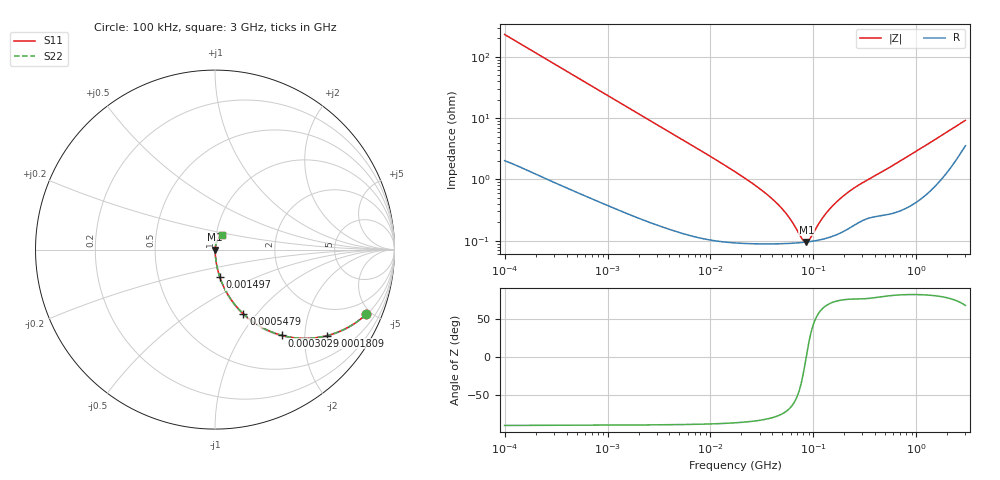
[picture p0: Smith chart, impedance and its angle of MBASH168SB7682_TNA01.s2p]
! MBASH168SB7682_TNA01  S-PARAMETER MODEL  ( Standard Model )
! Model Generated by TAIYO YUDEN Corporation (http://www.ty-top.com)
! Version 1.0
! TAIYO YUDEN Control No. 220601
! Copyright(c) 2013 TAIYO YUDEN CO.,LTD. All Rights Reserved.
! Product Description (link to TY-COMPAS)
! https://ds.yuden.co.jp/TYCOMPAS/or/detail?pn=MBASH168SB7682KTNA01&u=M
! Products Name : Multilayer Ceramic Capacitors
! Characteristics :
!  Capacitance : 6800 [pF] , Rated Voltage : 100 [V] , TCC : X7R
!  Case Size : 1.6 x 0.8 / 0.063 x 0.031 [mm/inch] , Thickness : 0.8 / 0.031 [mm/inch]
!  (Conditions: Temperature = 25 [degC] , DC Bias Voltage = 0 [V])
! External Node Assignments :
!  1  o---| |---o  2
! GND o---------o GND
! Frequency Range : 100kHz  -  3GHz  [ 401 STEP ]
# MHZ S RI R 50
! Freq[MHz].  S11 Real  S11 Imag  S21 Real  S21 Imag  S12 Real  S12 Imag  S22 Real  S22 Imag
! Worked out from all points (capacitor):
!   401 points, 100 kHz to 3 GHz, reference 50 ohm
!   read as one part in series: C = 6.84 nF near 105.3 kHz
!   lowest |Z| = 95.1 mohm at 85.61 MHz (marker M1)
!   series resonance near 85.27 MHz, so ESL is about 510 pH
!   S11 on the Smith chart (normalised r, x): 100 kHz: 1.04, -4.64; 180.9 kHz: 1.03, -2.58; 302.9 kHz: 1.02, -1.54; 547.9 kHz: 1.01, -0.86; 1.497 MHz: 1.01, -0.32; 3 GHz: 1.07, +0.17
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0.1  0.8413 -0.361  0.1587 0.361  0.1587 0.361  0.8413 -0.361
0.129398  0.7615 -0.4215  0.2385 0.4215  0.2385 0.4215  0.7615 -0.4215
0.180898  0.6228 -0.4796  0.3772 0.4796  0.3772 0.4796  0.6228 -0.4796
0.302894  0.3748 -0.4783  0.6252 0.4783  0.6252 0.4783  0.3748 -0.4783
0.54793  0.1585 -0.3586  0.8415 0.3586  0.8415 0.3586  0.1585 -0.3586
0.562235  0.152 -0.3523  0.848 0.3523  0.848 0.3523  0.152 -0.3523
0.871356  0.0715 -0.2501  0.9285 0.2501  0.9285 0.2501  0.0715 -0.2501
1.497078  0.027 -0.1535  0.973 0.1535  0.973 0.1535  0.027 -0.1535
3.161081  0.00736 -0.0747  0.9926 0.0747  0.9926 0.0747  0.00736 -0.0747
17.7727  0.00108 -0.0129  0.9989 0.0129  0.9989 0.0129  0.00108 -0.0129
30.53531  0.000933 -0.00687  0.9991 0.00687  0.9991 0.00687  0.000933 -0.00687
43.80277  0.000904 -0.00404  0.9991 0.00404  0.9991 0.00404  0.000904 -0.00404
58.15973  0.000907 -0.00221  0.9991 0.00221  0.9991 0.00221  0.000907 -0.00221
77.22239  0.000933 -0.00056  0.9991 0.00056  0.9991 0.00056  0.000933 -0.00056
85.60801  0.00095 2.25e-05  0.999 -2.25e-05  0.999 -2.25e-05  0.00095 2.25e-05
90.13636  0.00096 0.000313  0.999 -0.000313  0.999 -0.000313  0.00096 0.000313
97.38194  0.000979 0.000751  0.999 -0.000751  0.999 -0.000751  0.000979 0.000751
129.3002  0.00108 0.00241  0.9989 -0.00241  0.9989 -0.00241  0.00108 0.00241
180.7614  0.00134 0.0046  0.9987 -0.0046  0.9987 -0.0046  0.00134 0.0046
266.0711  0.00196 0.00754  0.998 -0.00754  0.998 -0.00754  0.00196 0.00754
547.5153  0.00293 0.0153  0.9971 -0.0153  0.9971 -0.0153  0.00293 0.0153
3000  0.0407 0.0787  0.9593 -0.0787  0.9593 -0.0787  0.0407 0.0787
